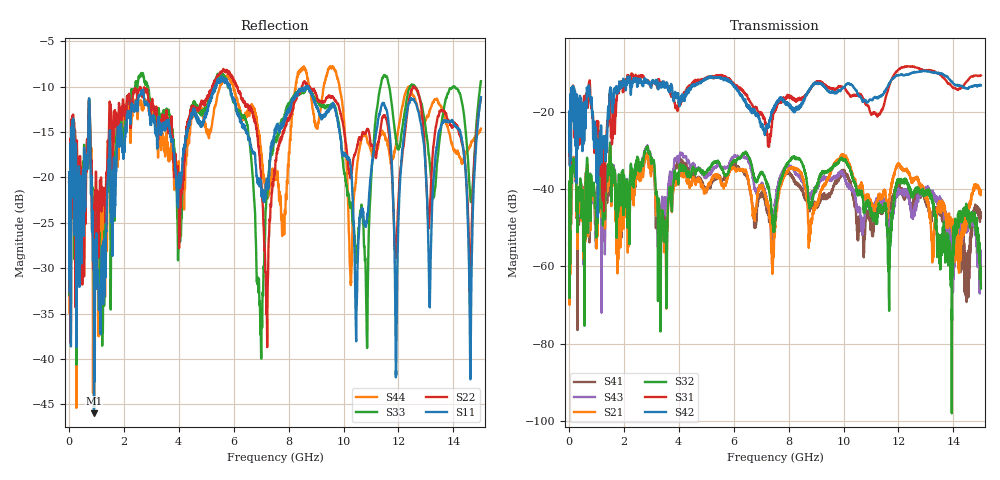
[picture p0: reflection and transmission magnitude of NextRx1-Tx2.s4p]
! FILE: N:\QM 2007\Prüfprotokolle\Highspeed\Konfektionierte Ltg\L45593-D106\D30\8216\0002\Next\NextRx1-Tx2.s4p
# MHz S DB R 50.00
! FREQ  S11  S12  S13  S14
!  S21  S22  S23  S24
!  S31  S32  S33  S34
!  S41  S42  S43  S44
!  DB  ANG  DB  ANG  DB  ANG  DB  ANG
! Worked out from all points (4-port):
!   2999 points, 10 MHz to 15 GHz, reference 50 ohm
!   strongest paths, dB at 10 MHz, 3.755 GHz, 7.505 GHz, 11.26 GHz, 15 GHz:
!     S42: -25.6, -13.4, -18.5, -16.4, -13.1
!     S31: -24.8, -15.3, -19.8, -20.7, -10.5
!     S32: -54.3, -45.8, -46.9, -44.9, -65.7
!     S21: -50.0, -45.4, -49.4, -42.4, -40.3
!     S43: -39.0, -38.6, -43.4, -43.6, -65.6
!     S41: -42.0, -39.3, -47.3, -44.8, -47.1
!   lowest |S11| = -46.0 dB at 915 MHz (marker M1), VSWR 1.01, Z = 50.3 + j0.403 ohm
!   |S11| at or under -10 dB: start of sweep to 5.329 GHz; 5.856 GHz to 8.621 GHz (2.765 GHz wide, 38.2 % of centre); 8.708 GHz to end of sweep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
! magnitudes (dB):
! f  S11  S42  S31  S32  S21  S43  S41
! 10 MHz  -19.4  -25.6  -24.8  -54.3  -50.0  -39.0  -42.0
! 160 MHz  -13.8  -13.9  -13.6  -35.0  -34.7  -35.3  -35.4
! 915 MHz  -46.0  -27.4  -24.4  -39.4  -39.6  -40.5  -41.3
! 7.43 GHz  -15.9  -19.7  -21.4  -48.5  -58.9  -50.7  -49.8
! 9.95 GHz  -17.5  -14.0  -13.7  -32.1  -31.0  -35.9  -35.4
! 14.62 GHz  -42.2  -13.4  -11.0  -47.9  -44.2  -48.6  -55.0
! 15 GHz  -11.1  -13.1  -10.5  -65.7  -40.3  -65.6  -47.1
